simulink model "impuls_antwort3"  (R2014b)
settings: Solver=ode4  StartTime=0.0  StopTime=20.0  MaxStep=0.001  RelTol=1e-3
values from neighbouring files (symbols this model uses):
  C = [0 1 0 0;0 0 0 1]    [impuls_antw_zustand_1.m]    (also in impuls_antwort_1.m = 1e-07; impuls_antwort_2.m = 1e-07; impuls_antwort_3.m = 1e-07; impuls_antwort_4.m = 1e-07)
  L = 0.01    [impuls_antwort_1.m]    (also in impuls_antwort_2.m; impuls_antwort_3.m; impuls_antwort_4.m; RLC_reihen_1.m)
  R = 50    [impuls_antwort_1.m]    (also in impuls_antwort_2.m; impuls_antwort_3.m; impuls_antwort_4.m; RLC_reihen_1.m)

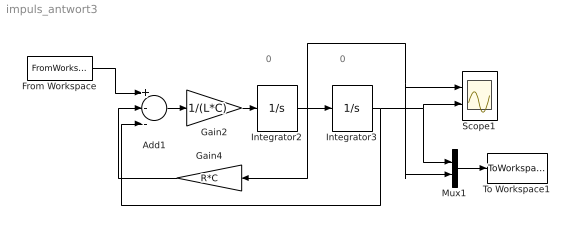
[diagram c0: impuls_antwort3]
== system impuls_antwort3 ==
  note: 0
  note: 0
  Add1 : Sum  Inputs=+--
  From Workspace : FromWorkspace  VariableName=[t', ug_puls']  SampleTime=0
  Gain2 : Gain  Gain=1/(L*C)
  Gain4 : Gain  Gain=R*C
  Integrator2 : Integrator
  Integrator3 : Integrator
  Mux1 : Mux  Inputs=2
  Scope1 : Scope  NumInputPorts=2
  To Workspace1 : ToWorkspace  VariableName=simout  SaveFormat=Timeseries  SampleTime=-1
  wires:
  Gain2/1 -> Integrator2/1
  Gain4/1 -> Add1/2
  From Workspace/1 -> Add1/1
  Integrator2/1 -> Mux1/2, Scope1/1, Gain4/1, Integrator3/1
  Integrator3/1 -> Mux1/1, Scope1/2, Add1/3
  Add1/1 -> Gain2/1
  Mux1/1 -> To Workspace1/1
